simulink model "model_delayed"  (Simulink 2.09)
settings: Solver=ode1  StartTime=0.0  StopTime=1  FixedStep=0.001  MaxStep=0.001  RelTol=1e-5  AbsTol=1e-5
undefined symbols (not defined in the file or in its folder): movedetect

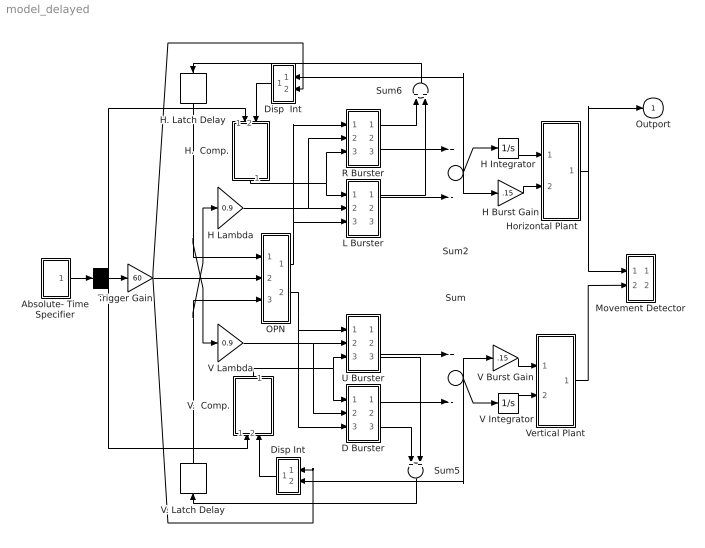
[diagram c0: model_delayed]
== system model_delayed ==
  . : Demux  Outputs=3
  Absolute- Time Specifier : Subsystem
  D Burster : Subsystem
  Disp  Int : Subsystem  Orientation=left
  Disp Int : Subsystem  Orientation=left
  H Burst Gain : Gain  Gain=.15
  H Integrator : Integrator  ExternalReset=none  InitialConditionSource=internal  InitialCondition=0  LimitOutput=off  UpperSaturationLimit=inf  LowerSaturationLimit=-inf  ShowSaturationPort=off  ShowStatePort=off  AbsoluteTolerance=auto
  H Lambda : Gain  Gain=0.9
  H.  Comp. : Subsystem  Orientation=down
  H. Latch Delay : TransportDelay  Orientation=down  DelayTime=.001  InitialInput=00  BufferSize=1024
  Horizontal Plant : Subsystem
  L Burster : Subsystem
  Movement Detector : Subsystem
  OPN : Subsystem
  R Burster : Subsystem
  Sum : Sum  Inputs=+-
  Sum2 : Sum  Inputs=+-
  Sum5 : Sum  Orientation=down  Inputs=++
  Sum6 : Sum  Orientation=up  Inputs=++
  Trigger Gain : Gain  Gain=60
  U Burster : Subsystem
  V Burst Gain : Gain  Gain=.15
  "V Integrator " : Integrator  ExternalReset=none  InitialConditionSource=internal  InitialCondition=0  LimitOutput=off  UpperSaturationLimit=inf  LowerSaturationLimit=-inf  ShowSaturationPort=off  ShowStatePort=off  AbsoluteTolerance=auto
  V Lambda : Gain  Gain=0.9
  V.  Comp. : Subsystem  Orientation=up
  V. Latch Delay : TransportDelay  Orientation=up  DelayTime=.001  InitialInput=00  BufferSize=1024
  Vertical Plant : Subsystem
  Outport : Outport  Port=1  InitialOutput=0
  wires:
  Trigger Gain/1 -> Disp Int/1(OPN Input), Disp  Int/2(Trigger), OPN/2(in_2)
  Horizontal Plant/1(out_1) -> Outport/1, Movement Detector/1(Horizontal Position)
  ./3 -> V.  Comp./1(in_4)
  Absolute- Time Specifier/1(out_1) -> ./1
  ./1 -> H.  Comp./1(in_1)
  ./2 -> Trigger Gain/1
  Vertical Plant/1(out_1) -> Movement Detector/2(Veritcal Position)
  H Integrator/1 -> Horizontal Plant/1(in_1)
  OPN/2(out_4) -> D Burster/3(in_3), U Burster/1(in_3)
  OPN/1(out_1) -> R Burster/1(in_3), L Burster/3(in_3)
  H. Latch Delay/1 -> V Lambda/1, OPN/1(in_1)
  V. Latch Delay/1 -> H Lambda/1, OPN/3(in_3)
  R Burster/1(out_2) -> Sum6/1
  Disp Int/1(out_1) -> V.  Comp./2(in_5)
  Disp  Int/1(out_1) -> H.  Comp./2(in_2)
  Sum5/1 -> V. Latch Delay/1
  Sum6/1 -> H. Latch Delay/1
  L Burster/1(out_1) -> Sum6/2
  V.  Comp./1(out_1) -> D Burster/1(in_1), U Burster/3(in_1)
  V Lambda/1 -> D Burster/2(in_2), U Burster/2(in_2)
  D Burster/2(out_2) -> Sum/2
  D Burster/3(out_3) -> Sum5/1
  U Burster/2(out_3) -> Sum/1
  U Burster/3(out_4) -> Sum5/2
  H Lambda/1 -> R Burster/2(in_2), L Burster/2(in_2)
  R Burster/2(out_3) -> Sum2/1
  L Burster/2(out_2) -> Sum2/2
  H.  Comp./1(out_1) -> R Burster/3(in_1), L Burster/1(in_1)
  Sum/1 -> Disp Int/2(BURST Input), "V Integrator "/1, V Burst Gain/1
  "V Integrator "/1 -> Vertical Plant/2(in_2)
  V Burst Gain/1 -> Vertical Plant/1(in_1)
  Sum2/1 -> Disp  Int/1(MLB Input), H Burst Gain/1, H Integrator/1
  H Burst Gain/1 -> Horizontal Plant/2(in_2)

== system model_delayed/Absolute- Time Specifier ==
  "Horizontal Specification " : FromWorkspace  VariableName=hspec
  Mux : Mux  Inputs=3
  Trigger : FromWorkspace  VariableName=trigspec
  Vertical Specification : FromWorkspace  VariableName=vspec
  out_1 : Outport  Port=1  InitialOutput=0
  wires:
  Mux/1 -> out_1/1
  Trigger/1 -> Mux/2
  "Horizontal Specification "/1 -> Mux/1
  Vertical Specification/1 -> Mux/3

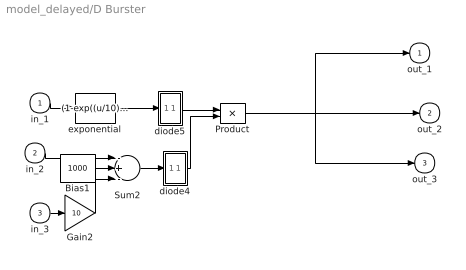
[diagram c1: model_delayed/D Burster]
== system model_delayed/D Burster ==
  in_1 : Inport  Port=1  PortWidth=-1  SampleTime=-1
  in_2 : Inport  Port=2  PortWidth=-1  SampleTime=-1
  in_3 : Inport  Port=3  PortWidth=-1  SampleTime=-1
  Bias1 : Constant  Value=1000
  Gain2 : Gain  Gain=10
  Product : Product  Inputs=2
  Sum2 : Sum  Inputs=-+-
  diode4 : Subsystem
  diode5 : Subsystem
  exponential : Fcn  Expr=(1-exp((u/10)))
  out_1 : Outport  Port=1  InitialOutput=0
  out_2 : Outport  Port=2  InitialOutput=0
  out_3 : Outport  Port=3  InitialOutput=0
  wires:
  in_1/1 -> exponential/1
  Bias1/1 -> Sum2/2
  in_2/1 -> Sum2/1
  in_3/1 -> Gain2/1
  Gain2/1 -> Sum2/3
  Sum2/1 -> diode4/1(in_1)
  diode4/1(out_1) -> Product/2
  exponential/1 -> diode5/1(in_1)
  diode5/1(out_1) -> Product/1
  Product/1 -> out_1/1, out_2/1, out_3/1

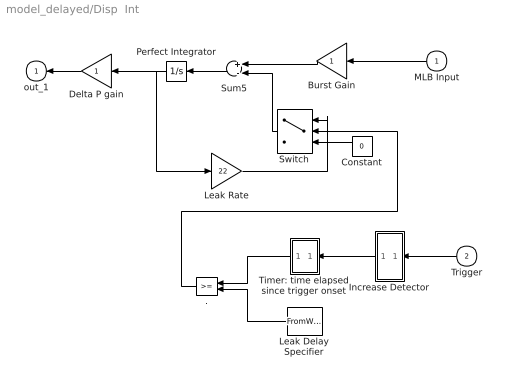
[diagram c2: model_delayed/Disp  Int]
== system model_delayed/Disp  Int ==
  MLB Input : Inport  Orientation=left  Port=1  PortWidth=-1  SampleTime=-1
  Trigger : Inport  Orientation=left  Port=2  PortWidth=-1  SampleTime=-1
  . : RelationalOperator  Orientation=left  Operator=>=
  Burst Gain : Gain  Orientation=left  Gain=1
  Constant : Constant  Orientation=left  Value=0
  Delta P gain : Gain  Orientation=left  Gain=1
  Increase Detector : Subsystem  Orientation=left
  Leak Delay Specifier : FromWorkspace  Orientation=left  VariableName=delay
  Leak Rate : Gain  Gain=22
  Perfect Integrator : Integrator  Orientation=left  ExternalReset=none  InitialConditionSource=internal  InitialCondition=0  LimitOutput=off  UpperSaturationLimit=inf  LowerSaturationLimit=-inf  ShowSaturationPort=off  ShowStatePort=off  AbsoluteTolerance=auto
  Sum5 : Sum  Orientation=left  Inputs=+-
  Switch : Switch  Orientation=left  Threshold=1
  Timer: time elapsed since trigger onset : Subsystem  Orientation=left
  out_1 : Outport  Orientation=left  Port=1  InitialOutput=0
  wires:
  ./1 -> Switch/2
  Leak Delay Specifier/1 -> ./2
  Timer: time elapsed since trigger onset/1(time) -> ./1
  Increase Detector/1(out_1) -> Timer: time elapsed since trigger onset/1(reset)
  Trigger/1 -> Increase Detector/1(Signal)
  Switch/1 -> Sum5/2
  Constant/1 -> Switch/3
  Leak Rate/1 -> Switch/1
  Perfect Integrator/1 -> Leak Rate/1, Delta P gain/1
  MLB Input/1 -> Burst Gain/1
  Burst Gain/1 -> Sum5/1
  Delta P gain/1 -> out_1/1
  Sum5/1 -> Perfect Integrator/1

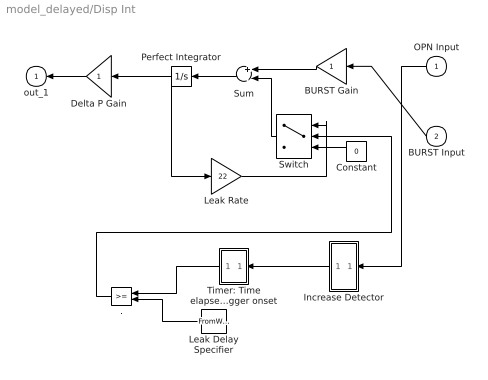
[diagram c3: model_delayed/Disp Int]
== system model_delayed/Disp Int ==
  OPN Input : Inport  Orientation=left  Port=1  PortWidth=-1  SampleTime=-1
  BURST Input : Inport  Orientation=left  Port=2  PortWidth=-1  SampleTime=-1
  . : RelationalOperator  Orientation=left  Operator=>=
  BURST Gain : Gain  Orientation=left  Gain=1
  Constant : Constant  Orientation=left  Value=0
  Delta P Gain : Gain  Orientation=left  Gain=1
  Increase Detector : Subsystem  Orientation=left
  Leak Delay Specifier : FromWorkspace  Orientation=left  VariableName=delay
  Leak Rate : Gain  Gain=22
  Perfect Integrator : Integrator  Orientation=left  ExternalReset=none  InitialConditionSource=internal  InitialCondition=0  LimitOutput=off  UpperSaturationLimit=inf  LowerSaturationLimit=-inf  ShowSaturationPort=off  ShowStatePort=off  AbsoluteTolerance=auto
  Sum : Sum  Orientation=left  Inputs=+-
  Switch : Switch  Orientation=left  Threshold=1
  Timer: Time elapsed since trigger onset : Subsystem  Orientation=left
  out_1 : Outport  Orientation=left  Port=1  InitialOutput=0
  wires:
  Timer: Time elapsed since trigger onset/1(time) -> ./1
  Increase Detector/1(out_1) -> Timer: Time elapsed since trigger onset/1(reset)
  Leak Delay Specifier/1 -> ./2
  ./1 -> Switch/2
  OPN Input/1 -> Increase Detector/1(Signal)
  BURST Input/1 -> BURST Gain/1
  Sum/1 -> Perfect Integrator/1
  Perfect Integrator/1 -> Delta P Gain/1, Leak Rate/1
  Delta P Gain/1 -> out_1/1
  BURST Gain/1 -> Sum/1
  Leak Rate/1 -> Switch/1
  Constant/1 -> Switch/3
  Switch/1 -> Sum/2

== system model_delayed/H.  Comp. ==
  in_1 : Inport  Port=1  PortWidth=-1  SampleTime=-1
  in_2 : Inport  Port=2  PortWidth=-1  SampleTime=-1
  Sum : Sum  Inputs=+-
  out_1 : Outport  Port=1  InitialOutput=0
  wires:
  in_2/1 -> Sum/2
  in_1/1 -> Sum/1
  Sum/1 -> out_1/1

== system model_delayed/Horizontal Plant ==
  in_1 : Inport  Orientation=left  Port=1  PortWidth=-1  SampleTime=-1
  in_2 : Inport  Orientation=left  Port=2  PortWidth=-1  SampleTime=-1
  Transfer Fcn1 : TransferFcn  Orientation=left  Numerator=[1]  Denominator=[.0018 .162 1]
  to Plant : Sum  Orientation=left  Inputs=++
  out_1 : Outport  Orientation=left  Port=1  InitialOutput=0
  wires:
  Transfer Fcn1/1 -> out_1/1
  in_2/1 -> to Plant/2
  in_1/1 -> to Plant/1
  to Plant/1 -> Transfer Fcn1/1

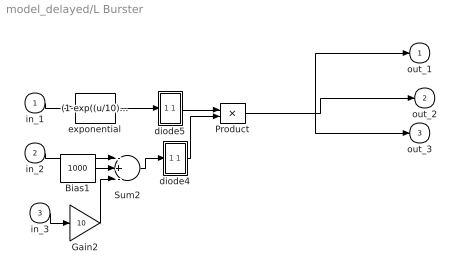
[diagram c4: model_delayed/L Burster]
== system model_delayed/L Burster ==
  in_1 : Inport  Port=1  PortWidth=-1  SampleTime=-1
  in_2 : Inport  Port=2  PortWidth=-1  SampleTime=-1
  in_3 : Inport  Port=3  PortWidth=-1  SampleTime=-1
  Bias1 : Constant  Value=1000
  Gain2 : Gain  Gain=10
  Product : Product  Inputs=2
  Sum2 : Sum  Inputs=-+-
  diode4 : Subsystem
  diode5 : Subsystem
  exponential : Fcn  Expr=(1-exp((u/10)))
  out_1 : Outport  Port=1  InitialOutput=0
  out_2 : Outport  Port=2  InitialOutput=0
  out_3 : Outport  Port=3  InitialOutput=0
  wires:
  Product/1 -> out_3/1, out_2/1, out_1/1
  diode5/1(out_1) -> Product/1
  exponential/1 -> diode5/1(in_1)
  diode4/1(out_1) -> Product/2
  Sum2/1 -> diode4/1(in_1)
  Gain2/1 -> Sum2/3
  in_3/1 -> Gain2/1
  in_2/1 -> Sum2/1
  Bias1/1 -> Sum2/2
  in_1/1 -> exponential/1

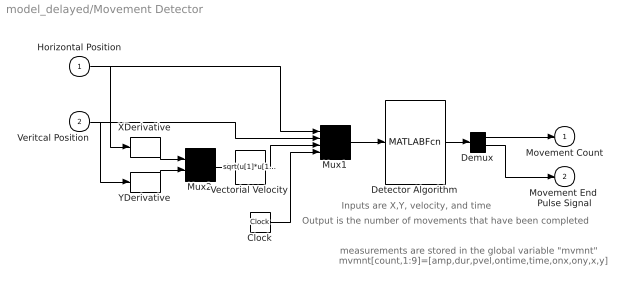
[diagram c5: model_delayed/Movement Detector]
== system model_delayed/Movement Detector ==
  note: mvmnt[count,1:9]=[amp,dur,pvel,ontime,time,onx,ony,x,y]
  note: measurements are stored in the global variable "mvmnt"
  note: Inputs are X,Y, velocity, and time
  note: Output is the number of movements that have been completed
  Horizontal Position : Inport  Port=1  PortWidth=-1  SampleTime=-1
  Veritcal Position : Inport  Port=2  PortWidth=-1  SampleTime=-1
  Clock : Clock
  Demux : Demux  Outputs=2
  Detector Algorithm : MATLABFcn  MATLABFcn=movedetect(u(1),u(2),u(3),u(4))  OutputWidth=2
  Mux1 : Mux  Inputs=4
  Mux2 : Mux  Inputs=2
  Vectorial Velocity : Fcn  Expr=sqrt(u[1]*u[1]+u[2]*u[2])
  XDerivative : Derivative
  YDerivative : Derivative
  Movement Count : Outport  Port=1  InitialOutput=0
  Movement End  Pulse Signal : Outport  Port=2  InitialOutput=0
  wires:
  Demux/2 -> Movement End  Pulse Signal/1
  Demux/1 -> Movement Count/1
  Detector Algorithm/1 -> Demux/1
  Horizontal Position/1 -> XDerivative/1, Mux1/1
  Veritcal Position/1 -> YDerivative/1, Mux1/2
  Vectorial Velocity/1 -> Mux1/3
  Clock/1 -> Mux1/4
  Mux2/1 -> Vectorial Velocity/1
  XDerivative/1 -> Mux2/1
  YDerivative/1 -> Mux2/2
  Mux1/1 -> Detector Algorithm/1

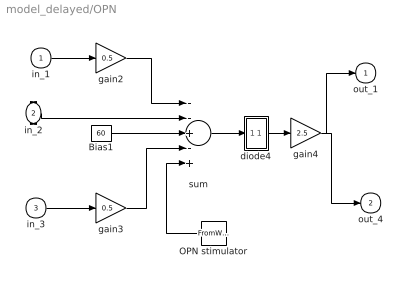
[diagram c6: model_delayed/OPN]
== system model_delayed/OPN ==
  in_1 : Inport  Port=1  PortWidth=-1  SampleTime=-1
  in_2 : Inport  Port=2  PortWidth=-1  SampleTime=-1
  in_3 : Inport  Port=3  PortWidth=-1  SampleTime=-1
  Bias1 : Constant  Value=60
  OPN stimulator : FromWorkspace  Orientation=left  VariableName=stimulate
  diode4 : Subsystem
  gain2 : Gain  Gain=0.5
  gain3 : Gain  Gain=0.5
  gain4 : Gain  Gain=2.5
  sum : Sum  Inputs=--+-+
  out_1 : Outport  Port=1  InitialOutput=0
  out_4 : Outport  Port=2  InitialOutput=0
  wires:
  OPN stimulator/1 -> sum/5
  gain4/1 -> out_4/1, out_1/1
  diode4/1(out_1) -> gain4/1
  gain3/1 -> sum/4
  in_3/1 -> gain3/1
  gain2/1 -> sum/1
  in_1/1 -> gain2/1
  Bias1/1 -> sum/3
  in_2/1 -> sum/2
  sum/1 -> diode4/1(in_1)

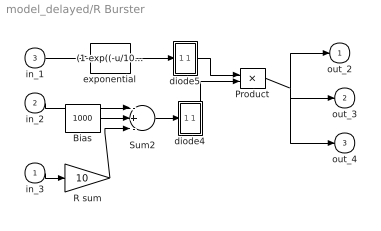
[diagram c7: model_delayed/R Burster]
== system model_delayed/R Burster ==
  in_3 : Inport  Port=1  PortWidth=-1  SampleTime=-1
  in_2 : Inport  Port=2  PortWidth=-1  SampleTime=-1
  in_1 : Inport  Port=3  PortWidth=-1  SampleTime=-1
  Bias : Constant  Value=1000
  Product : Product  Inputs=2
  R sum : Gain  Gain=10
  Sum2 : Sum  Inputs=-+-
  diode4 : Subsystem
  diode5 : Subsystem
  exponential : Fcn  Expr=(1-exp((-u/10)))
  out_2 : Outport  Port=1  InitialOutput=0
  out_3 : Outport  Port=2  InitialOutput=0
  out_4 : Outport  Port=3  InitialOutput=0
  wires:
  diode5/1(out_1) -> Product/1
  exponential/1 -> diode5/1(in_1)
  diode4/1(out_1) -> Product/2
  Sum2/1 -> diode4/1(in_1)
  in_1/1 -> exponential/1
  in_2/1 -> Sum2/1
  Bias/1 -> Sum2/2
  Product/1 -> out_2/1, out_4/1, out_3/1
  in_3/1 -> R sum/1
  R sum/1 -> Sum2/3

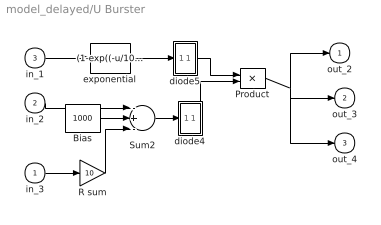
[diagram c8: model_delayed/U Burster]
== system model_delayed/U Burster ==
  in_3 : Inport  Port=1  PortWidth=-1  SampleTime=-1
  in_2 : Inport  Port=2  PortWidth=-1  SampleTime=-1
  in_1 : Inport  Port=3  PortWidth=-1  SampleTime=-1
  Bias : Constant  Value=1000
  Product : Product  Inputs=2
  R sum : Gain  Gain=10
  Sum2 : Sum  Inputs=-+-
  diode4 : Subsystem
  diode5 : Subsystem
  exponential : Fcn  Expr=(1-exp((-u/10)))
  out_2 : Outport  Port=1  InitialOutput=0
  out_3 : Outport  Port=2  InitialOutput=0
  out_4 : Outport  Port=3  InitialOutput=0
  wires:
  diode5/1(out_1) -> Product/1
  exponential/1 -> diode5/1(in_1)
  diode4/1(out_1) -> Product/2
  Sum2/1 -> diode4/1(in_1)
  in_1/1 -> exponential/1
  in_2/1 -> Sum2/1
  Bias/1 -> Sum2/2
  Product/1 -> out_2/1, out_4/1, out_3/1
  in_3/1 -> R sum/1
  R sum/1 -> Sum2/3

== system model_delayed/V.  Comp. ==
  in_4 : Inport  Port=1  PortWidth=-1  SampleTime=-1
  in_5 : Inport  Port=2  PortWidth=-1  SampleTime=-1
  Sum : Sum  Inputs=-+
  out_1 : Outport  Port=1  InitialOutput=0
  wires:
  in_4/1 -> Sum/2
  in_5/1 -> Sum/1
  Sum/1 -> out_1/1

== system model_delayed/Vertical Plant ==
  in_1 : Inport  Orientation=left  Port=1  PortWidth=-1  SampleTime=-1
  in_2 : Inport  Orientation=left  Port=2  PortWidth=-1  SampleTime=-1
  Transfer Fcn1 : TransferFcn  Orientation=left  Numerator=[1]  Denominator=[.0018 .162 1]
  to Plant : Sum  Orientation=left  Inputs=++
  out_1 : Outport  Orientation=left  Port=1  InitialOutput=0
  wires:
  Transfer Fcn1/1 -> out_1/1
  in_2/1 -> to Plant/2
  in_1/1 -> to Plant/1
  to Plant/1 -> Transfer Fcn1/1

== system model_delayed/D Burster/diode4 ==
  in_1 : Inport  Port=1  PortWidth=-1  SampleTime=-1
  Switch : Switch  Threshold=0
  diode1 : Constant  Value=0
  out_1 : Outport  Port=1  InitialOutput=0
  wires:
  in_1/1 -> Switch/2, Switch/1
  Switch/1 -> out_1/1
  diode1/1 -> Switch/3

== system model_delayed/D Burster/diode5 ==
  in_1 : Inport  Port=1  PortWidth=-1  SampleTime=-1
  Switch : Switch  Threshold=0
  diode1 : Constant  Value=0
  out_1 : Outport  Port=1  InitialOutput=0
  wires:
  in_1/1 -> Switch/2, Switch/1
  Switch/1 -> out_1/1
  diode1/1 -> Switch/3

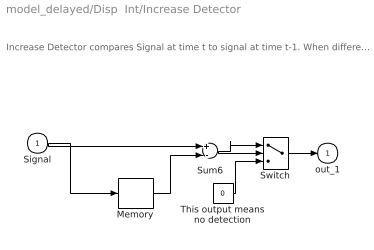
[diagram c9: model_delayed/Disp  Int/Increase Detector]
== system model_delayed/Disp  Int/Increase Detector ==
  note: Increase Detector compares Signal at time t to signal at time t-1. When difference is greater than the Switch threshold, it outputs the difference (positive), 0 otherwise.
  Signal : Inport  Port=1  PortWidth=-1  SampleTime=-1
  Memory : Memory  X0=0  InheritSampleTime=off
  Sum6 : Sum  Inputs=+-
  Switch : Switch  Threshold=0.001
  This output means no detection : Constant  Value=0
  out_1 : Outport  Port=1  InitialOutput=0
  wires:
  This output means no detection/1 -> Switch/3
  Sum6/1 -> Switch/1, Switch/2
  Memory/1 -> Sum6/2
  Signal/1 -> Memory/1, Sum6/1
  Switch/1 -> out_1/1

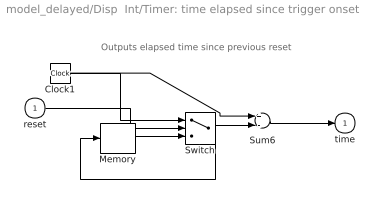
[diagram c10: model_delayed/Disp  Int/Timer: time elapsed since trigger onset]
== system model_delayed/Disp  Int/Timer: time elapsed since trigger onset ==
  note: Outputs elapsed time since previous reset
  reset : Inport  Port=1  PortWidth=-1  SampleTime=-1
  Clock1 : Clock
  Memory : Memory  X0=0  InheritSampleTime=off
  Sum6 : Sum  Inputs=+-
  Switch : Switch  Threshold=0.001
  time : Outport  Port=1  InitialOutput=0
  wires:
  Switch/1 -> Memory/1, Sum6/2
  Memory/1 -> Switch/3
  reset/1 -> Switch/2
  Clock1/1 -> Switch/1, Sum6/1
  Sum6/1 -> time/1

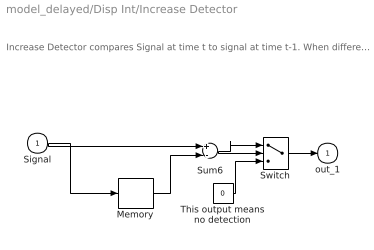
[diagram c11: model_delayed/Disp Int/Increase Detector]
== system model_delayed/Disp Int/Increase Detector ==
  note: Increase Detector compares Signal at time t to signal at time t-1. When difference is greater than the Switch threshold, it outputs the difference (positive), 0 otherwise.
  Signal : Inport  Port=1  PortWidth=-1  SampleTime=-1
  Memory : Memory  X0=0  InheritSampleTime=off
  Sum6 : Sum  Inputs=+-
  Switch : Switch  Threshold=0.001
  This output means no detection : Constant  Value=0
  out_1 : Outport  Port=1  InitialOutput=0
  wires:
  Signal/1 -> Sum6/1, Memory/1
  Switch/1 -> out_1/1
  Memory/1 -> Sum6/2
  Sum6/1 -> Switch/2, Switch/1
  This output means no detection/1 -> Switch/3

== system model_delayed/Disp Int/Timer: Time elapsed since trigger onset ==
  note: Outputs elapsed time since previous reset
  reset : Inport  Port=1  PortWidth=-1  SampleTime=-1
  Clock1 : Clock
  Memory : Memory  X0=0  InheritSampleTime=off
  Sum6 : Sum  Inputs=+-
  Switch : Switch  Threshold=0.001
  time : Outport  Port=1  InitialOutput=0
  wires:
  Switch/1 -> Sum6/2, Memory/1
  Sum6/1 -> time/1
  Clock1/1 -> Sum6/1, Switch/1
  reset/1 -> Switch/2
  Memory/1 -> Switch/3

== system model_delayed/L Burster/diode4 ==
  in_1 : Inport  Port=1  PortWidth=-1  SampleTime=-1
  Switch : Switch  Threshold=0
  diode1 : Constant  Value=0
  out_1 : Outport  Port=1  InitialOutput=0
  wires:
  diode1/1 -> Switch/3
  Switch/1 -> out_1/1
  in_1/1 -> Switch/2, Switch/1

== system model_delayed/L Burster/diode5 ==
  in_1 : Inport  Port=1  PortWidth=-1  SampleTime=-1
  Switch : Switch  Threshold=0
  diode1 : Constant  Value=0
  out_1 : Outport  Port=1  InitialOutput=0
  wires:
  diode1/1 -> Switch/3
  Switch/1 -> out_1/1
  in_1/1 -> Switch/2, Switch/1

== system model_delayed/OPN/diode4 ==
  in_1 : Inport  Port=1  PortWidth=-1  SampleTime=-1
  Switch : Switch  Threshold=0
  diode1 : Constant  Value=0
  out_1 : Outport  Port=1  InitialOutput=0
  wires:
  in_1/1 -> Switch/2, Switch/1
  Switch/1 -> out_1/1
  diode1/1 -> Switch/3

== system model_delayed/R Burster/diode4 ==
  in_1 : Inport  Port=1  PortWidth=-1  SampleTime=-1
  Switch : Switch  Threshold=0
  diode1 : Constant  Value=0
  out_1 : Outport  Port=1  InitialOutput=0
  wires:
  in_1/1 -> Switch/2, Switch/1
  Switch/1 -> out_1/1
  diode1/1 -> Switch/3

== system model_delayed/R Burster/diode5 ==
  in_1 : Inport  Port=1  PortWidth=-1  SampleTime=-1
  Switch : Switch  Threshold=0
  diode1 : Constant  Value=0
  out_1 : Outport  Port=1  InitialOutput=0
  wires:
  diode1/1 -> Switch/3
  Switch/1 -> out_1/1
  in_1/1 -> Switch/2, Switch/1

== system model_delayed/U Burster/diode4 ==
  in_1 : Inport  Port=1  PortWidth=-1  SampleTime=-1
  Switch : Switch  Threshold=0
  diode1 : Constant  Value=0
  out_1 : Outport  Port=1  InitialOutput=0
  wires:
  in_1/1 -> Switch/2, Switch/1
  Switch/1 -> out_1/1
  diode1/1 -> Switch/3

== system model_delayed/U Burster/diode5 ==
  in_1 : Inport  Port=1  PortWidth=-1  SampleTime=-1
  Switch : Switch  Threshold=0
  diode1 : Constant  Value=0
  out_1 : Outport  Port=1  InitialOutput=0
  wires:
  diode1/1 -> Switch/3
  Switch/1 -> out_1/1
  in_1/1 -> Switch/2, Switch/1
